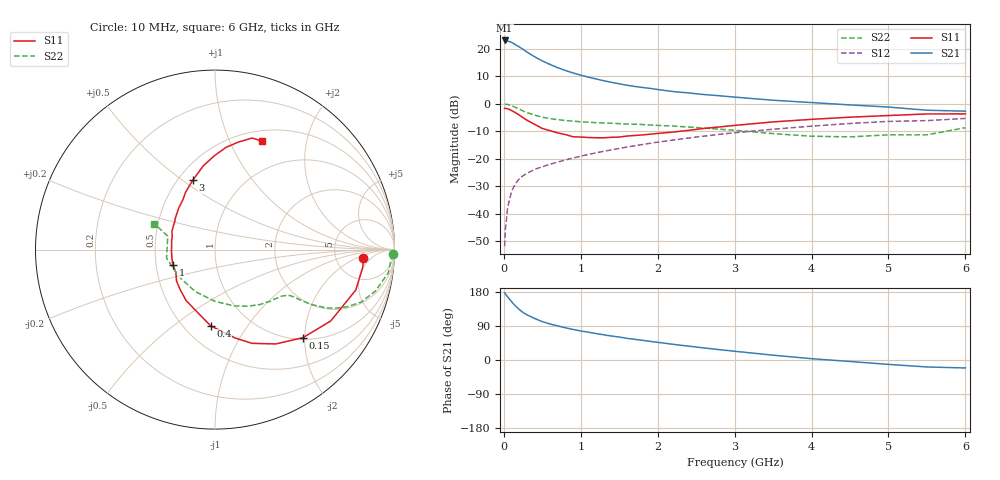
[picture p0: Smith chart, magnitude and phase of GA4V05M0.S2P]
! Infineon Technologies  Discrete & RF Semiconductors
! BF775
! Si NPN RF Bipolar Junction Transistor in SOT23
! VCE = 4 V  IC = 5 mA
! Common Emitter S-Parameters:  May  1996
# GHz  S  MA  R  50
!  f  S11  S21  S12  S22
! GHz  MAG  ANG  MAG  ANG  MAG  ANG  MAG  ANG
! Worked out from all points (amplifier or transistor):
!   36 points, 10 MHz to 6 GHz, reference 50 ohm
!   highest |S21| = 23.0 dB at 10 MHz (marker M1)
!   |S21| within 3 dB of that: start of sweep to 237.3 MHz
!   unconditionally stable (mu >= 1): 809.6 MHz to 3.36 GHz
!   at 250 MHz: K = 0.48, MSG = 22.9 dB, |S12| = -26.1 dB
!   at 1.4 GHz: K = 1.12, MAG = 10.1 dB, |S12| = -16.7 dB
!   at 6 GHz: K = 0.95, MSG = 1.3 dB, |S12| = -5.3 dB
!   lowest NFmin = 1.50 dB at 450 MHz
!   S11 on the Smith chart (normalised r, x): 10 MHz: 10, -3; 150 MHz: 1.04, -1.96; 400 MHz: 0.67, -0.69; 1 GHz: 0.61, -0.11; 3 GHz: 0.59, +0.55; 6 GHz: 0.63, +1.33
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0.01  0.8274 -3.3  14.19 177.3  0.0026 86.9  0.9926 -1.5
0.02  0.8296 -6.6  13.99 174.2  0.0052 86.4  0.9828 -3.1
0.05  0.8162 -16.0  13.82 166.5  0.0132 80.8  0.9741 -7.6
0.1  0.7574 -31.7  13.16 154.1  0.0255 73.5  0.9242 -14.4
0.15  0.6931 -45.1  11.88 142.6  0.0354 67.5  0.865 -19.8
0.2  0.6253 -57.2  10.86 133.5  0.0435 63.8  0.8025 -23.4
0.25  0.5613 -68.5  9.782 125.4  0.0497 60.5  0.7412 -26.2
0.3  0.5053 -77.1  8.737 119.3  0.0549 58.4  0.6941 -27.8
0.4  0.4251 -93.3  7.189 109.7  0.0645 56.4  0.6244 -29.5
0.5  0.3573 -107.2  6.021 101.3  0.0722 56.4  0.5731 -30.3
0.6  0.3259 -119.7  5.198 95.1  0.08 56.2  0.5392 -30.7
0.8  0.2768 -140.7  4.038 85.1  0.0957 57.0  0.498 -31.3
1  0.2497 -160.5  3.321 76.7  0.1118 57.7  0.4734 -32.6
1.1  0.2446 -169.2  3.057 73.3  0.1207 58.0  0.4643 -33.6
1.3  0.2422 175.7  2.632 66.4  0.1379 58.0  0.4495 -35.6
1.6  0.2604 157.3  2.18 57.2  0.1641 57.0  0.4308 -39.8
2.2  0.3078 130.9  1.674 41.4  0.2202 53.7  0.3961 -50.6
3  0.406 107.7  1.327 23.1  0.2988 46.2  0.3315 -71.3
3.5  0.4702 98.1  1.164 12.7  0.3463 40.5  0.288 -90.1
4.5  0.5731 83.8  0.957 -3.9  0.44 27.8  0.2512 -143.5
5.5  0.6557 71.5  0.766 -18.4  0.4969 12.8  0.2736 164.1
6  0.6581 66.3  0.737 -21.0  0.5435 8.6  0.369 156.8
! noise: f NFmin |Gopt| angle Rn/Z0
0.45  1.5  0.28  29  0.34
0.9  1.8  0.25  59  0.34
